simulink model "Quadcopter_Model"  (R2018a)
settings: Solver=VariableStepAuto  StartTime=0.0  StopTime=runtime  FixedStep=0.001  RelTol=1e-3
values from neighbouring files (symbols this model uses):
  delta_T = [ 0,  0,  9.404e-04 ]    [modelParameters.m]    (also in rich_params.m = [ 0,  0,  1.176e-04 ])
  g = 9.81    [modelParameters.m]    (also in rich_params.m)
  height_controlled_o = (((Rm*If        + (((omega0_o * 2 * Rm * Kv * Kq      * Kd + 1)^2) - 1)/(4* Rm*Kv^2*Kq      * Kd))/Vb)*(Pmax - Pmin) + Pmin)    [modelParameters.m]    (also in rich_params.m)
  If = 0.3836    [modelParameters.m]    (also in rich_params.m = 0.39)
  Jreq = 4.2012e-05    [modelParameters.m]    (also in rich_params.m = 1.376e-05)
  Jxx = 0.0110    (= 0.011)    [modelParameters.m]    (also in rich_params.m = 0.0081)
  Jyy = 0.0116    [modelParameters.m]    (also in rich_params.m = 0.0074)
  Jzz = 0.0223    [modelParameters.m]    (also in rich_params.m = 0.0135)
  Kd = 1.4852e-07    [modelParameters.m]    (also in rich_params.m = 5.194e-07)
  Kh = 3.4574e-04    (= 0.00034574)    [modelParameters.m]    (also in rich_params.m)
  Kq = 96.3422    [modelParameters.m]    (also in rich_params.m = 110)
  Kt = 1.2007e-05    [modelParameters.m]    (also in rich_params.m = 7.3956e-06)
  Kv = 96.3422    [modelParameters.m]    (also in rich_params.m = 110)
  m = 1.216    [modelParameters.m]    (also in rich_params.m = 0.656)
  omega0_o = sqrt((m*g)/(4*Kt))    [modelParameters.m]    (also in rich_params.m)
  omega1_o = sqrt((m*g)/(4*Kt))    [modelParameters.m]    (also in rich_params.m)
  omega2_o = sqrt((m*g)/(4*Kt))    [modelParameters.m]    (also in rich_params.m)
  omega3_o = sqrt((m*g)/(4*Kt))    [modelParameters.m]    (also in rich_params.m)
  pitch_o = 0    [modelParameters.m]    (also in rich_params.m)
  pitchrate_o = 0    [modelParameters.m]    (also in rich_params.m)
  Pmax = 1    [modelParameters.m]    (also in rich_params.m)
  Pmin = 0    [modelParameters.m]    (also in rich_params.m)
  r_oc = [ 0 ; 0 ; 0 ]    [modelParameters.m]    (also in rich_params.m)
  rhx = 0.16    [modelParameters.m]    (also in rich_params.m = 0.115)
  rhy = 0.16    [modelParameters.m]    (also in rich_params.m = 0.115)
  rhz = 0.03    [modelParameters.m]    (also in rich_params.m = 0.04)
  Rm = 0.235    [modelParameters.m]    (also in rich_params.m = 0.19)
  roll_o = 0    [modelParameters.m]    (also in rich_params.m)
  rollrate_o = 0    [modelParameters.m]    (also in rich_params.m)
  signal_mixer = [ 1, -1, -1, -1    [modelParameters.m]    (also in rich_params.m)
  Tc = 0.01    [modelParameters.m]    (also in rich_params.m)
  Tq = 0.005    [modelParameters.m]    (also in rich_params.m)
  Vb = 12.3    [modelParameters.m]    (also in rich_params.m = 11.4)
  x_controlled_o = 0    [modelParameters.m]    (also in rich_params.m)
  x_o = 0    [modelParameters.m]    (also in rich_params.m)
  x_vel_o = 0    [modelParameters.m]    (also in rich_params.m)
  y_controlled_o = 0    [modelParameters.m]    (also in rich_params.m)
  y_o = 0    [modelParameters.m]    (also in rich_params.m)
  y_vel_o = 0    [modelParameters.m]    (also in rich_params.m)
  yaw_controlled_o = 0    [modelParameters.m]    (also in rich_params.m)
  yaw_o = 0    [modelParameters.m]    (also in rich_params.m)
  yawrate_o = 0    [modelParameters.m]    (also in rich_params.m)
  z_o = 0    [modelParameters.m]    (also in rich_params.m)
  z_vel_o = 0    [modelParameters.m]    (also in rich_params.m)
undefined symbols (not defined in the file or in its folder): lqr_K
libraries: simulink x16, Derivative x13, dsparch4 x3, vrlib x1
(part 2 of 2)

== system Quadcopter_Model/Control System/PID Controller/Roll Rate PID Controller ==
  rollrate_error : Inport
  rollrate : Inport  Port=2
  Add : Sum  Inputs=+-
  Discrete D Controller : Derivative/Discrete D Controller  Kd=Kd  a=a
  Discrete PI Controller : simulink/Continuous/PID Controller  Controller=PI  TimeDomain=Discrete-time  SampleTime=Ts  IntegratorMethod=Forward Euler  FilterMethod=Forward Euler  Form=Parallel  UseFilter=on  ControllerParametersSource=internal  P=Kp  I=Ki  D=0  N=100  InitialConditionSource=internal  InitialConditionForIntegrator=0  InitialConditionForFilter=0  ExternalReset=none  LimitOutput=off  UpperSaturationLimit=inf  LowerSaturationLimit=-inf  LinearizeAsGain=off  AntiWindupMode=none  Kb=1  TrackingMode=off  Kt=1  PParamMin=[]  PParamMax=[]  IParamMin=[]  IParamMax=[]  DParamMin=[]  DParamMax=[]  NParamMin=[]  NParamMax=[]  KbParamMin=[]  KbParamMax=[]  KtParamMin=[]  KtParamMax=[]  POutMin=[]  POutMax=[]  IOutMin=[]  IOutMax=[]  DOutMin=[]  DOutMax=[]  NOutMin=[]  NOutMax=[]  KbOutMin=[]  KbOutMax=[]  KtOutMin=[]  KtOutMax=[]  IntegratorOutMin=[]  IntegratorOutMax=[]  FilterOutMin=[]  FilterOutMax=[]  SumOutMin=[]  SumOutMax=[]  SumI1OutMin=[]  SumI1OutMax=[]  SumI2OutMin=[]  SumI2OutMax=[]  SumI3OutMin=[]  SumI3OutMax=[]  SumDOutMin=[]  SumDOutMax=[]  SaturationOutMin=[]  SaturationOutMax=[]  IntegratorContinuousStateAttributes=''  IntegratorStateMustResolveToSignalObject=off  IntegratorRTWStateStorageClass=Auto  FilterContinuousStateAttributes=''  FilterStateMustResolveToSignalObject=off  FilterRTWStateStorageClass=Auto  DifferentiatorICPrevScaledInput=0  DifferentiatorOutMin=[]  DifferentiatorOutMax=[]  FilterDiffOutCoefMin=[]  FilterDiffOutCoefMax=[]  SumDenOutMin=[]  SumDenOutMax=[]  SumNumOutMin=[]  SumNumOutMax=[]  ReciprocalOutMin=[]  ReciprocalOutMax=[]  DivideOutMin=[]  DivideOutMax=[]  TunerSelectOption=Transfer Function Based (PID Tuner App)
  y_motor_command : Outport
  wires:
  rollrate/1 -> Discrete D Controller/1
  rollrate_error/1 -> Discrete PI Controller/1
  Discrete PI Controller/1 -> Add/1
  Discrete D Controller/1 -> Add/2
  Add/1 -> y_motor_command/1

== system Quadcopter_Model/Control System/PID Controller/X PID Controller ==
  x_error : Inport
  x_pos : Inport  Port=2
  Add : Sum  Inputs=+-
  Discrete D Controller : Derivative/Discrete D Controller  Kd=Kd  a=a
  Discrete PI Controller : simulink/Continuous/PID Controller  Controller=PI  TimeDomain=Discrete-time  SampleTime=Ts  IntegratorMethod=Forward Euler  FilterMethod=Forward Euler  Form=Parallel  UseFilter=on  ControllerParametersSource=internal  P=Kp  I=Ki  D=0  N=100  InitialConditionSource=internal  InitialConditionForIntegrator=0  InitialConditionForFilter=0  ExternalReset=none  LimitOutput=off  UpperSaturationLimit=inf  LowerSaturationLimit=-inf  LinearizeAsGain=off  AntiWindupMode=none  Kb=1  TrackingMode=off  Kt=1  PParamMin=[]  PParamMax=[]  IParamMin=[]  IParamMax=[]  DParamMin=[]  DParamMax=[]  NParamMin=[]  NParamMax=[]  KbParamMin=[]  KbParamMax=[]  KtParamMin=[]  KtParamMax=[]  POutMin=[]  POutMax=[]  IOutMin=[]  IOutMax=[]  DOutMin=[]  DOutMax=[]  NOutMin=[]  NOutMax=[]  KbOutMin=[]  KbOutMax=[]  KtOutMin=[]  KtOutMax=[]  IntegratorOutMin=[]  IntegratorOutMax=[]  FilterOutMin=[]  FilterOutMax=[]  SumOutMin=[]  SumOutMax=[]  SumI1OutMin=[]  SumI1OutMax=[]  SumI2OutMin=[]  SumI2OutMax=[]  SumI3OutMin=[]  SumI3OutMax=[]  SumDOutMin=[]  SumDOutMax=[]  SaturationOutMin=[]  SaturationOutMax=[]  IntegratorContinuousStateAttributes=''  IntegratorStateMustResolveToSignalObject=off  IntegratorRTWStateStorageClass=Auto  FilterContinuousStateAttributes=''  FilterStateMustResolveToSignalObject=off  FilterRTWStateStorageClass=Auto  DifferentiatorICPrevScaledInput=0  DifferentiatorOutMin=[]  DifferentiatorOutMax=[]  FilterDiffOutCoefMin=[]  FilterDiffOutCoefMax=[]  SumDenOutMin=[]  SumDenOutMax=[]  SumNumOutMin=[]  SumNumOutMax=[]  ReciprocalOutMin=[]  ReciprocalOutMax=[]  DivideOutMin=[]  DivideOutMax=[]  TunerSelectOption=Transfer Function Based (PID Tuner App)
  pitch_setpoint : Outport
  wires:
  x_pos/1 -> Discrete D Controller/1
  x_error/1 -> Discrete PI Controller/1
  Discrete PI Controller/1 -> Add/1
  Discrete D Controller/1 -> Add/2
  Add/1 -> pitch_setpoint/1

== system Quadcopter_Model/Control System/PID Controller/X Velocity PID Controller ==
  x_vel_error : Inport
  x_vel : Inport  Port=2
  Add : Sum  Inputs=+-
  Discrete D Controller : Derivative/Discrete D Controller  Kd=Kd  a=a
  Discrete PI Controller : simulink/Continuous/PID Controller  Controller=PI  TimeDomain=Discrete-time  SampleTime=Ts  IntegratorMethod=Forward Euler  FilterMethod=Forward Euler  Form=Parallel  UseFilter=on  ControllerParametersSource=internal  P=Kp  I=Ki  D=0  N=100  InitialConditionSource=internal  InitialConditionForIntegrator=0  InitialConditionForFilter=0  ExternalReset=none  LimitOutput=off  UpperSaturationLimit=inf  LowerSaturationLimit=-inf  LinearizeAsGain=off  AntiWindupMode=none  Kb=1  TrackingMode=off  Kt=1  PParamMin=[]  PParamMax=[]  IParamMin=[]  IParamMax=[]  DParamMin=[]  DParamMax=[]  NParamMin=[]  NParamMax=[]  KbParamMin=[]  KbParamMax=[]  KtParamMin=[]  KtParamMax=[]  POutMin=[]  POutMax=[]  IOutMin=[]  IOutMax=[]  DOutMin=[]  DOutMax=[]  NOutMin=[]  NOutMax=[]  KbOutMin=[]  KbOutMax=[]  KtOutMin=[]  KtOutMax=[]  IntegratorOutMin=[]  IntegratorOutMax=[]  FilterOutMin=[]  FilterOutMax=[]  SumOutMin=[]  SumOutMax=[]  SumI1OutMin=[]  SumI1OutMax=[]  SumI2OutMin=[]  SumI2OutMax=[]  SumI3OutMin=[]  SumI3OutMax=[]  SumDOutMin=[]  SumDOutMax=[]  SaturationOutMin=[]  SaturationOutMax=[]  IntegratorContinuousStateAttributes=''  IntegratorStateMustResolveToSignalObject=off  IntegratorRTWStateStorageClass=Auto  FilterContinuousStateAttributes=''  FilterStateMustResolveToSignalObject=off  FilterRTWStateStorageClass=Auto  DifferentiatorICPrevScaledInput=0  DifferentiatorOutMin=[]  DifferentiatorOutMax=[]  FilterDiffOutCoefMin=[]  FilterDiffOutCoefMax=[]  SumDenOutMin=[]  SumDenOutMax=[]  SumNumOutMin=[]  SumNumOutMax=[]  ReciprocalOutMin=[]  ReciprocalOutMax=[]  DivideOutMin=[]  DivideOutMax=[]  TunerSelectOption=Transfer Function Based (PID Tuner App)
  pitch_setpoint : Outport
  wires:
  x_vel/1 -> Discrete D Controller/1
  x_vel_error/1 -> Discrete PI Controller/1
  Discrete PI Controller/1 -> Add/1
  Discrete D Controller/1 -> Add/2
  Add/1 -> pitch_setpoint/1

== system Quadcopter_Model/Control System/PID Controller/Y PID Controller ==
  y_error : Inport
  y_pos : Inport  Port=2
  Add : Sum  Inputs=+-
  Discrete D Controller : Derivative/Discrete D Controller  Kd=Kd  a=a
  Discrete PI Controller : simulink/Continuous/PID Controller  Controller=PI  TimeDomain=Discrete-time  SampleTime=Ts  IntegratorMethod=Forward Euler  FilterMethod=Forward Euler  Form=Parallel  UseFilter=on  ControllerParametersSource=internal  P=Kp  I=Ki  D=0  N=100  InitialConditionSource=internal  InitialConditionForIntegrator=0  InitialConditionForFilter=0  ExternalReset=none  LimitOutput=off  UpperSaturationLimit=inf  LowerSaturationLimit=-inf  LinearizeAsGain=off  AntiWindupMode=none  Kb=1  TrackingMode=off  Kt=1  PParamMin=[]  PParamMax=[]  IParamMin=[]  IParamMax=[]  DParamMin=[]  DParamMax=[]  NParamMin=[]  NParamMax=[]  KbParamMin=[]  KbParamMax=[]  KtParamMin=[]  KtParamMax=[]  POutMin=[]  POutMax=[]  IOutMin=[]  IOutMax=[]  DOutMin=[]  DOutMax=[]  NOutMin=[]  NOutMax=[]  KbOutMin=[]  KbOutMax=[]  KtOutMin=[]  KtOutMax=[]  IntegratorOutMin=[]  IntegratorOutMax=[]  FilterOutMin=[]  FilterOutMax=[]  SumOutMin=[]  SumOutMax=[]  SumI1OutMin=[]  SumI1OutMax=[]  SumI2OutMin=[]  SumI2OutMax=[]  SumI3OutMin=[]  SumI3OutMax=[]  SumDOutMin=[]  SumDOutMax=[]  SaturationOutMin=[]  SaturationOutMax=[]  IntegratorContinuousStateAttributes=''  IntegratorStateMustResolveToSignalObject=off  IntegratorRTWStateStorageClass=Auto  FilterContinuousStateAttributes=''  FilterStateMustResolveToSignalObject=off  FilterRTWStateStorageClass=Auto  DifferentiatorICPrevScaledInput=0  DifferentiatorOutMin=[]  DifferentiatorOutMax=[]  FilterDiffOutCoefMin=[]  FilterDiffOutCoefMax=[]  SumDenOutMin=[]  SumDenOutMax=[]  SumNumOutMin=[]  SumNumOutMax=[]  ReciprocalOutMin=[]  ReciprocalOutMax=[]  DivideOutMin=[]  DivideOutMax=[]  TunerSelectOption=Transfer Function Based (PID Tuner App)
  roll_setpoint : Outport
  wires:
  y_pos/1 -> Discrete D Controller/1
  y_error/1 -> Discrete PI Controller/1
  Discrete PI Controller/1 -> Add/1
  Discrete D Controller/1 -> Add/2
  Add/1 -> roll_setpoint/1

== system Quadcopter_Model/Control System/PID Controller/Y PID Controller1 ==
  y_error : Inport
  y_pos : Inport  Port=2
  Add : Sum  Inputs=+-
  Discrete D Controller : Derivative/Discrete D Controller  Kd=Kd  a=a
  Discrete PI Controller : simulink/Continuous/PID Controller  Controller=PI  TimeDomain=Discrete-time  SampleTime=Ts  IntegratorMethod=Forward Euler  FilterMethod=Forward Euler  Form=Parallel  UseFilter=on  ControllerParametersSource=internal  P=Kp  I=Ki  D=0  N=100  InitialConditionSource=internal  InitialConditionForIntegrator=0  InitialConditionForFilter=0  ExternalReset=none  LimitOutput=off  UpperSaturationLimit=inf  LowerSaturationLimit=-inf  LinearizeAsGain=off  AntiWindupMode=none  Kb=1  TrackingMode=off  Kt=1  PParamMin=[]  PParamMax=[]  IParamMin=[]  IParamMax=[]  DParamMin=[]  DParamMax=[]  NParamMin=[]  NParamMax=[]  KbParamMin=[]  KbParamMax=[]  KtParamMin=[]  KtParamMax=[]  POutMin=[]  POutMax=[]  IOutMin=[]  IOutMax=[]  DOutMin=[]  DOutMax=[]  NOutMin=[]  NOutMax=[]  KbOutMin=[]  KbOutMax=[]  KtOutMin=[]  KtOutMax=[]  IntegratorOutMin=[]  IntegratorOutMax=[]  FilterOutMin=[]  FilterOutMax=[]  SumOutMin=[]  SumOutMax=[]  SumI1OutMin=[]  SumI1OutMax=[]  SumI2OutMin=[]  SumI2OutMax=[]  SumI3OutMin=[]  SumI3OutMax=[]  SumDOutMin=[]  SumDOutMax=[]  SaturationOutMin=[]  SaturationOutMax=[]  IntegratorContinuousStateAttributes=''  IntegratorStateMustResolveToSignalObject=off  IntegratorRTWStateStorageClass=Auto  FilterContinuousStateAttributes=''  FilterStateMustResolveToSignalObject=off  FilterRTWStateStorageClass=Auto  DifferentiatorICPrevScaledInput=0  DifferentiatorOutMin=[]  DifferentiatorOutMax=[]  FilterDiffOutCoefMin=[]  FilterDiffOutCoefMax=[]  SumDenOutMin=[]  SumDenOutMax=[]  SumNumOutMin=[]  SumNumOutMax=[]  ReciprocalOutMin=[]  ReciprocalOutMax=[]  DivideOutMin=[]  DivideOutMax=[]  TunerSelectOption=Transfer Function Based (PID Tuner App)
  y_vel_setpoint : Outport
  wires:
  y_pos/1 -> Discrete D Controller/1
  y_error/1 -> Discrete PI Controller/1
  Discrete PI Controller/1 -> Add/1
  Discrete D Controller/1 -> Add/2
  Add/1 -> y_vel_setpoint/1

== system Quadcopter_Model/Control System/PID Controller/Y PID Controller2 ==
  x_error : Inport
  x_pos : Inport  Port=2
  Add : Sum  Inputs=+-
  Discrete D Controller : Derivative/Discrete D Controller  Kd=Kd  a=a
  Discrete PI Controller : simulink/Continuous/PID Controller  Controller=PI  TimeDomain=Discrete-time  SampleTime=Ts  IntegratorMethod=Forward Euler  FilterMethod=Forward Euler  Form=Parallel  UseFilter=on  ControllerParametersSource=internal  P=Kp  I=Ki  D=0  N=100  InitialConditionSource=internal  InitialConditionForIntegrator=0  InitialConditionForFilter=0  ExternalReset=none  LimitOutput=off  UpperSaturationLimit=inf  LowerSaturationLimit=-inf  LinearizeAsGain=off  AntiWindupMode=none  Kb=1  TrackingMode=off  Kt=1  PParamMin=[]  PParamMax=[]  IParamMin=[]  IParamMax=[]  DParamMin=[]  DParamMax=[]  NParamMin=[]  NParamMax=[]  KbParamMin=[]  KbParamMax=[]  KtParamMin=[]  KtParamMax=[]  POutMin=[]  POutMax=[]  IOutMin=[]  IOutMax=[]  DOutMin=[]  DOutMax=[]  NOutMin=[]  NOutMax=[]  KbOutMin=[]  KbOutMax=[]  KtOutMin=[]  KtOutMax=[]  IntegratorOutMin=[]  IntegratorOutMax=[]  FilterOutMin=[]  FilterOutMax=[]  SumOutMin=[]  SumOutMax=[]  SumI1OutMin=[]  SumI1OutMax=[]  SumI2OutMin=[]  SumI2OutMax=[]  SumI3OutMin=[]  SumI3OutMax=[]  SumDOutMin=[]  SumDOutMax=[]  SaturationOutMin=[]  SaturationOutMax=[]  IntegratorContinuousStateAttributes=''  IntegratorStateMustResolveToSignalObject=off  IntegratorRTWStateStorageClass=Auto  FilterContinuousStateAttributes=''  FilterStateMustResolveToSignalObject=off  FilterRTWStateStorageClass=Auto  DifferentiatorICPrevScaledInput=0  DifferentiatorOutMin=[]  DifferentiatorOutMax=[]  FilterDiffOutCoefMin=[]  FilterDiffOutCoefMax=[]  SumDenOutMin=[]  SumDenOutMax=[]  SumNumOutMin=[]  SumNumOutMax=[]  ReciprocalOutMin=[]  ReciprocalOutMax=[]  DivideOutMin=[]  DivideOutMax=[]  TunerSelectOption=Transfer Function Based (PID Tuner App)
  x_vel_setpoint : Outport
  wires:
  x_pos/1 -> Discrete D Controller/1
  x_error/1 -> Discrete PI Controller/1
  Discrete PI Controller/1 -> Add/1
  Discrete D Controller/1 -> Add/2
  Add/1 -> x_vel_setpoint/1

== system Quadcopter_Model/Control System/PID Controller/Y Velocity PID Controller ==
  y_error : Inport
  y_pos : Inport  Port=2
  Add : Sum  Inputs=+-
  Discrete D Controller : Derivative/Discrete D Controller  Kd=Kd  a=a
  Discrete PI Controller : simulink/Continuous/PID Controller  Controller=PI  TimeDomain=Discrete-time  SampleTime=Ts  IntegratorMethod=Forward Euler  FilterMethod=Forward Euler  Form=Parallel  UseFilter=on  ControllerParametersSource=internal  P=Kp  I=Ki  D=0  N=100  InitialConditionSource=internal  InitialConditionForIntegrator=0  InitialConditionForFilter=0  ExternalReset=none  LimitOutput=off  UpperSaturationLimit=inf  LowerSaturationLimit=-inf  LinearizeAsGain=off  AntiWindupMode=none  Kb=1  TrackingMode=off  Kt=1  PParamMin=[]  PParamMax=[]  IParamMin=[]  IParamMax=[]  DParamMin=[]  DParamMax=[]  NParamMin=[]  NParamMax=[]  KbParamMin=[]  KbParamMax=[]  KtParamMin=[]  KtParamMax=[]  POutMin=[]  POutMax=[]  IOutMin=[]  IOutMax=[]  DOutMin=[]  DOutMax=[]  NOutMin=[]  NOutMax=[]  KbOutMin=[]  KbOutMax=[]  KtOutMin=[]  KtOutMax=[]  IntegratorOutMin=[]  IntegratorOutMax=[]  FilterOutMin=[]  FilterOutMax=[]  SumOutMin=[]  SumOutMax=[]  SumI1OutMin=[]  SumI1OutMax=[]  SumI2OutMin=[]  SumI2OutMax=[]  SumI3OutMin=[]  SumI3OutMax=[]  SumDOutMin=[]  SumDOutMax=[]  SaturationOutMin=[]  SaturationOutMax=[]  IntegratorContinuousStateAttributes=''  IntegratorStateMustResolveToSignalObject=off  IntegratorRTWStateStorageClass=Auto  FilterContinuousStateAttributes=''  FilterStateMustResolveToSignalObject=off  FilterRTWStateStorageClass=Auto  DifferentiatorICPrevScaledInput=0  DifferentiatorOutMin=[]  DifferentiatorOutMax=[]  FilterDiffOutCoefMin=[]  FilterDiffOutCoefMax=[]  SumDenOutMin=[]  SumDenOutMax=[]  SumNumOutMin=[]  SumNumOutMax=[]  ReciprocalOutMin=[]  ReciprocalOutMax=[]  DivideOutMin=[]  DivideOutMax=[]  TunerSelectOption=Transfer Function Based (PID Tuner App)
  roll_setpoint : Outport
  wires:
  y_pos/1 -> Discrete D Controller/1
  y_error/1 -> Discrete PI Controller/1
  Discrete PI Controller/1 -> Add/1
  Discrete D Controller/1 -> Add/2
  Add/1 -> roll_setpoint/1

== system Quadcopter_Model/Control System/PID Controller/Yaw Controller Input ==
  note: 1) Add Subsystem or Model blocks as valid variant choices. 2) You cannot connect blocks at this level. At simulation, connectivity is automatically determined, based on the active variant and port name matching.
  yaw_error_model : Inport
  yaw_angle_model : Inport  Port=2
  Feedback : Subsystem  VariantControl=logAnalysisToggle==0
  yaw error : Subsystem  VariantControl=logAnalysisToggle==1
  yaw_error : Outport
  yaw_angle : Outport  Port=2

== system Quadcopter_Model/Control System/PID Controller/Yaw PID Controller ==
  yaw_error : Inport
  yaw_angle : Inport  Port=2
  Add : Sum  Inputs=+-
  Discrete D Controller : Derivative/Discrete D Controller  Kd=Kd  a=a
  Discrete PI Controller : simulink/Continuous/PID Controller  Controller=PI  TimeDomain=Discrete-time  SampleTime=Ts  IntegratorMethod=Forward Euler  FilterMethod=Forward Euler  Form=Parallel  UseFilter=on  ControllerParametersSource=internal  P=Kp  I=Ki  D=0  N=100  InitialConditionSource=internal  InitialConditionForIntegrator=0  InitialConditionForFilter=0  ExternalReset=none  LimitOutput=off  UpperSaturationLimit=inf  LowerSaturationLimit=-inf  LinearizeAsGain=off  AntiWindupMode=none  Kb=1  TrackingMode=off  Kt=1  PParamMin=[]  PParamMax=[]  IParamMin=[]  IParamMax=[]  DParamMin=[]  DParamMax=[]  NParamMin=[]  NParamMax=[]  KbParamMin=[]  KbParamMax=[]  KtParamMin=[]  KtParamMax=[]  POutMin=[]  POutMax=[]  IOutMin=[]  IOutMax=[]  DOutMin=[]  DOutMax=[]  NOutMin=[]  NOutMax=[]  KbOutMin=[]  KbOutMax=[]  KtOutMin=[]  KtOutMax=[]  IntegratorOutMin=[]  IntegratorOutMax=[]  FilterOutMin=[]  FilterOutMax=[]  SumOutMin=[]  SumOutMax=[]  SumI1OutMin=[]  SumI1OutMax=[]  SumI2OutMin=[]  SumI2OutMax=[]  SumI3OutMin=[]  SumI3OutMax=[]  SumDOutMin=[]  SumDOutMax=[]  SaturationOutMin=[]  SaturationOutMax=[]  IntegratorContinuousStateAttributes=''  IntegratorStateMustResolveToSignalObject=off  IntegratorRTWStateStorageClass=Auto  FilterContinuousStateAttributes=''  FilterStateMustResolveToSignalObject=off  FilterRTWStateStorageClass=Auto  DifferentiatorICPrevScaledInput=0  DifferentiatorOutMin=[]  DifferentiatorOutMax=[]  FilterDiffOutCoefMin=[]  FilterDiffOutCoefMax=[]  SumDenOutMin=[]  SumDenOutMax=[]  SumNumOutMin=[]  SumNumOutMax=[]  ReciprocalOutMin=[]  ReciprocalOutMax=[]  DivideOutMin=[]  DivideOutMax=[]  TunerSelectOption=Transfer Function Based (PID Tuner App)
  yawrate_setpoint : Outport
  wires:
  yaw_angle/1 -> Discrete D Controller/1
  yaw_error/1 -> Discrete PI Controller/1
  Discrete PI Controller/1 -> Add/1
  Discrete D Controller/1 -> Add/2
  Add/1 -> yawrate_setpoint/1

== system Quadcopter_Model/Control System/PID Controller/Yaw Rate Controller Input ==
  note: 1) Add Subsystem or Model blocks as valid variant choices. 2) You cannot connect blocks at this level. At simulation, connectivity is automatically determined, based on the active variant and port name matching.
  yawrate_error_model : Inport
  yawrate_model : Inport  Port=2
  Feedback : Subsystem  VariantControl=logAnalysisToggle==0
  yawrate error : Subsystem  VariantControl=logAnalysisToggle==1
  yawrate_error : Outport
  yawrate : Outport  Port=2

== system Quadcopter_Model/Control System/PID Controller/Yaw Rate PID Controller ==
  yawrate_error : Inport
  yawrate : Inport  Port=2
  Add : Sum  Inputs=+-
  Discrete D Controller : Derivative/Discrete D Controller  Kd=Kd  a=a
  Discrete PI Controller : simulink/Continuous/PID Controller  Controller=PI  TimeDomain=Discrete-time  SampleTime=Ts  IntegratorMethod=Forward Euler  FilterMethod=Forward Euler  Form=Parallel  UseFilter=on  ControllerParametersSource=internal  P=Kp  I=Ki  D=0  N=100  InitialConditionSource=internal  InitialConditionForIntegrator=0  InitialConditionForFilter=0  ExternalReset=none  LimitOutput=off  UpperSaturationLimit=inf  LowerSaturationLimit=-inf  LinearizeAsGain=off  AntiWindupMode=none  Kb=1  TrackingMode=off  Kt=1  PParamMin=[]  PParamMax=[]  IParamMin=[]  IParamMax=[]  DParamMin=[]  DParamMax=[]  NParamMin=[]  NParamMax=[]  KbParamMin=[]  KbParamMax=[]  KtParamMin=[]  KtParamMax=[]  POutMin=[]  POutMax=[]  IOutMin=[]  IOutMax=[]  DOutMin=[]  DOutMax=[]  NOutMin=[]  NOutMax=[]  KbOutMin=[]  KbOutMax=[]  KtOutMin=[]  KtOutMax=[]  IntegratorOutMin=[]  IntegratorOutMax=[]  FilterOutMin=[]  FilterOutMax=[]  SumOutMin=[]  SumOutMax=[]  SumI1OutMin=[]  SumI1OutMax=[]  SumI2OutMin=[]  SumI2OutMax=[]  SumI3OutMin=[]  SumI3OutMax=[]  SumDOutMin=[]  SumDOutMax=[]  SaturationOutMin=[]  SaturationOutMax=[]  IntegratorContinuousStateAttributes=''  IntegratorStateMustResolveToSignalObject=off  IntegratorRTWStateStorageClass=Auto  FilterContinuousStateAttributes=''  FilterStateMustResolveToSignalObject=off  FilterRTWStateStorageClass=Auto  DifferentiatorICPrevScaledInput=0  DifferentiatorOutMin=[]  DifferentiatorOutMax=[]  FilterDiffOutCoefMin=[]  FilterDiffOutCoefMax=[]  SumDenOutMin=[]  SumDenOutMax=[]  SumNumOutMin=[]  SumNumOutMax=[]  ReciprocalOutMin=[]  ReciprocalOutMax=[]  DivideOutMin=[]  DivideOutMax=[]  TunerSelectOption=Transfer Function Based (PID Tuner App)
  yaw_motor_command : Outport
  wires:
  yawrate/1 -> Discrete D Controller/1
  yawrate_error/1 -> Discrete PI Controller/1
  Discrete PI Controller/1 -> Add/1
  Discrete D Controller/1 -> Add/2
  Add/1 -> yaw_motor_command/1

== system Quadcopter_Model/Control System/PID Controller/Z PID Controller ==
  z_error : Inport
  z_pos : Inport  Port=2
  Add : Sum  Inputs=+-
  Discrete D Controller : Derivative/Discrete D Controller  Kd=Kd  a=a
  Discrete PI Controller : simulink/Continuous/PID Controller  Controller=PI  TimeDomain=Discrete-time  SampleTime=Ts  IntegratorMethod=Forward Euler  FilterMethod=Forward Euler  Form=Parallel  UseFilter=on  ControllerParametersSource=internal  P=Kp  I=Ki  D=0  N=100  InitialConditionSource=internal  InitialConditionForIntegrator=0  InitialConditionForFilter=0  ExternalReset=none  LimitOutput=off  UpperSaturationLimit=inf  LowerSaturationLimit=-inf  LinearizeAsGain=off  AntiWindupMode=none  Kb=1  TrackingMode=off  Kt=1  PParamMin=[]  PParamMax=[]  IParamMin=[]  IParamMax=[]  DParamMin=[]  DParamMax=[]  NParamMin=[]  NParamMax=[]  KbParamMin=[]  KbParamMax=[]  KtParamMin=[]  KtParamMax=[]  POutMin=[]  POutMax=[]  IOutMin=[]  IOutMax=[]  DOutMin=[]  DOutMax=[]  NOutMin=[]  NOutMax=[]  KbOutMin=[]  KbOutMax=[]  KtOutMin=[]  KtOutMax=[]  IntegratorOutMin=[]  IntegratorOutMax=[]  FilterOutMin=[]  FilterOutMax=[]  SumOutMin=[]  SumOutMax=[]  SumI1OutMin=[]  SumI1OutMax=[]  SumI2OutMin=[]  SumI2OutMax=[]  SumI3OutMin=[]  SumI3OutMax=[]  SumDOutMin=[]  SumDOutMax=[]  SaturationOutMin=[]  SaturationOutMax=[]  IntegratorContinuousStateAttributes=''  IntegratorStateMustResolveToSignalObject=off  IntegratorRTWStateStorageClass=Auto  FilterContinuousStateAttributes=''  FilterStateMustResolveToSignalObject=off  FilterRTWStateStorageClass=Auto  DifferentiatorICPrevScaledInput=0  DifferentiatorOutMin=[]  DifferentiatorOutMax=[]  FilterDiffOutCoefMin=[]  FilterDiffOutCoefMax=[]  SumDenOutMin=[]  SumDenOutMax=[]  SumNumOutMin=[]  SumNumOutMax=[]  ReciprocalOutMin=[]  ReciprocalOutMax=[]  DivideOutMin=[]  DivideOutMax=[]  TunerSelectOption=Transfer Function Based (PID Tuner App)
  z_motor_command : Outport
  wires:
  z_pos/1 -> Discrete D Controller/1
  z_error/1 -> Discrete PI Controller/1
  Discrete PI Controller/1 -> Add/1
  Discrete D Controller/1 -> Add/2
  Add/1 -> z_motor_command/1

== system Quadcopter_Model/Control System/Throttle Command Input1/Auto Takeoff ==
  height_controlled_o : Constant  Value=0.45  SampleTime=Tc
  z_command : Outport
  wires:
  height_controlled_o/1 -> z_command/1

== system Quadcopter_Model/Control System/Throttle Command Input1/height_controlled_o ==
  height_controlled_o : Constant  Value=height_controlled_o  SampleTime=Tc
  z_command : Outport
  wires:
  height_controlled_o/1 -> z_command/1

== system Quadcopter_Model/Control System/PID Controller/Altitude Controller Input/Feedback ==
  z_error_model : Inport
  z_position_model : Inport  Port=2
  z_error : Outport
  z_position : Outport  Port=2
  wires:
  z_error_model/1 -> z_error/1
  z_position_model/1 -> z_position/1

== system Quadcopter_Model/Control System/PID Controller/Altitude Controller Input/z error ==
  From Workspace1 : FromWorkspace  VariableName=z_position  SampleTime=Tc  Interpolate=off  OutputAfterFinalValue=Holding final value
  From Workspace6 : FromWorkspace  VariableName=z_error  SampleTime=Tc  Interpolate=off  OutputAfterFinalValue=Holding final value
  z_error : Outport
  z_position : Outport  Port=2
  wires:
  From Workspace6/1 -> z_error/1
  From Workspace1/1 -> z_position/1

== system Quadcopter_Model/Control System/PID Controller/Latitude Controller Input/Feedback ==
  x_error_model : Inport
  x_position_model : Inport  Port=2
  x_error : Outport
  x_position : Outport  Port=2
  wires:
  x_error_model/1 -> x_error/1
  x_position_model/1 -> x_position/1

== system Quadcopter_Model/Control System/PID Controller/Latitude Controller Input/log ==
  From Workspace : FromWorkspace  VariableName=x_error  SampleTime=Tc  Interpolate=off  OutputAfterFinalValue=Holding final value
  From Workspace1 : FromWorkspace  VariableName=x_position  SampleTime=Tc  Interpolate=off  OutputAfterFinalValue=Holding final value
  x_error : Outport
  x_position : Outport  Port=2
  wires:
  From Workspace/1 -> x_error/1
  From Workspace1/1 -> x_position/1

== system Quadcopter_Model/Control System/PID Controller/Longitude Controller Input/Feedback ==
  y_error_model : Inport
  y_position_model : Inport  Port=2
  y_error : Outport
  y_position : Outport  Port=2
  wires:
  y_error_model/1 -> y_error/1
  y_position_model/1 -> y_position/1

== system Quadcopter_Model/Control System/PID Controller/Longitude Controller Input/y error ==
  From Workspace1 : FromWorkspace  VariableName=y_position  SampleTime=Tc  Interpolate=off  OutputAfterFinalValue=Holding final value
  From Workspace3 : FromWorkspace  VariableName=y_error  SampleTime=Tc  Interpolate=off  OutputAfterFinalValue=Holding final value
  y_error : Outport
  y_position : Outport  Port=2
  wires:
  From Workspace3/1 -> y_error/1
  From Workspace1/1 -> y_position/1

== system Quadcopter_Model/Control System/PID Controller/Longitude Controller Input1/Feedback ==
  y_vel_error_model : Inport
  y_vel_model : Inport  Port=2
  y_vel_error : Outport
  y_vel : Outport  Port=2
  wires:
  y_vel_error_model/1 -> y_vel_error/1
  y_vel_model/1 -> y_vel/1

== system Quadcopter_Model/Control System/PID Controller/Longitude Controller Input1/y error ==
  From Workspace1 : FromWorkspace  VariableName=y_vel  SampleTime=Tc  Interpolate=off  OutputAfterFinalValue=Holding final value
  From Workspace3 : FromWorkspace  VariableName=y_vel_error  SampleTime=Tc  Interpolate=off  OutputAfterFinalValue=Holding final value
  y_vel_error : Outport
  y_vel : Outport  Port=2
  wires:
  From Workspace3/1 -> y_vel_error/1
  From Workspace1/1 -> y_vel/1

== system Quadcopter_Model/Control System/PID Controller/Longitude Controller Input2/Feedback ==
  x_vel_error_model : Inport
  x_vel_model : Inport  Port=2
  x_vel_error : Outport
  x_vel : Outport  Port=2
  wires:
  x_vel_error_model/1 -> x_vel_error/1
  x_vel_model/1 -> x_vel/1

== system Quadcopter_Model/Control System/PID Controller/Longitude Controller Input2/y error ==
  From Workspace1 : FromWorkspace  VariableName=x_vel  SampleTime=Tc  Interpolate=off  OutputAfterFinalValue=Holding final value
  From Workspace3 : FromWorkspace  VariableName=x_vel_error  SampleTime=Tc  Interpolate=off  OutputAfterFinalValue=Holding final value
  x_vel_error : Outport
  x_vel : Outport  Port=2
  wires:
  From Workspace3/1 -> x_vel_error/1
  From Workspace1/1 -> x_vel/1

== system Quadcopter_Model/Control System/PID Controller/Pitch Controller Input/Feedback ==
  pitch_error_model : Inport
  pitch_angle_model : Inport  Port=2
  pitch_error : Outport
  pitch_angle : Outport  Port=2
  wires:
  pitch_error_model/1 -> pitch_error/1
  pitch_angle_model/1 -> pitch_angle/1

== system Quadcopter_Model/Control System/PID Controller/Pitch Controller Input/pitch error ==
  From Workspace : FromWorkspace  VariableName=pitch_error  SampleTime=Tq  Interpolate=off  OutputAfterFinalValue=Holding final value
  From Workspace1 : FromWorkspace  VariableName=pitch_angle  SampleTime=Tq  Interpolate=off  OutputAfterFinalValue=Holding final value
  pitch_error : Outport
  pitch_angle : Outport  Port=2
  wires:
  From Workspace/1 -> pitch_error/1
  From Workspace1/1 -> pitch_angle/1

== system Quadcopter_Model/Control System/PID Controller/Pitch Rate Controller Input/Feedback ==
  pitchrate_error_model : Inport
  pitchrate_model : Inport  Port=2
  pitchrate_error : Outport
  pitchrate : Outport  Port=2
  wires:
  pitchrate_error_model/1 -> pitchrate_error/1
  pitchrate_model/1 -> pitchrate/1

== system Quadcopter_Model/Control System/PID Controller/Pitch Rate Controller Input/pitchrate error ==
  From Workspace1 : FromWorkspace  VariableName=pitchrate  SampleTime=Tq  Interpolate=off  OutputAfterFinalValue=Holding final value
  From Workspace2 : FromWorkspace  VariableName=pitchrate_error  SampleTime=Tq  Interpolate=off  OutputAfterFinalValue=Holding final value
  pitchrate_error : Outport
  pitchrate : Outport  Port=2
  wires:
  From Workspace2/1 -> pitchrate_error/1
  From Workspace1/1 -> pitchrate/1

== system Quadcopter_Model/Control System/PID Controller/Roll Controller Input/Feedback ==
  roll_error_model : Inport
  roll_angle_model : Inport  Port=2
  roll_error : Outport
  roll_angle : Outport  Port=2
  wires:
  roll_error_model/1 -> roll_error/1
  roll_angle_model/1 -> roll_angle/1

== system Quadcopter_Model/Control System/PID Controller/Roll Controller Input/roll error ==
  From Workspace1 : FromWorkspace  VariableName=roll_angle  SampleTime=Tq  Interpolate=off  OutputAfterFinalValue=Holding final value
  From Workspace4 : FromWorkspace  VariableName=roll_error  SampleTime=Tq  Interpolate=off  OutputAfterFinalValue=Holding final value
  roll_error : Outport
  roll_angle : Outport  Port=2
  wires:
  From Workspace4/1 -> roll_error/1
  From Workspace1/1 -> roll_angle/1

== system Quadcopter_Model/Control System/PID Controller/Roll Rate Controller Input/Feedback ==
  rollrate_error_model : Inport
  rollrate_model : Inport  Port=2
  rollrate_error : Outport
  rollrate : Outport  Port=2
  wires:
  rollrate_error_model/1 -> rollrate_error/1
  rollrate_model/1 -> rollrate/1

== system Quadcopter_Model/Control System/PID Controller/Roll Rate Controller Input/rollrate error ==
  From Workspace1 : FromWorkspace  VariableName=rollrate  SampleTime=Tq  Interpolate=off  OutputAfterFinalValue=Holding final value
  From Workspace5 : FromWorkspace  VariableName=rollrate_error  SampleTime=Tq  Interpolate=off  OutputAfterFinalValue=Holding final value
  rollrate_error : Outport
  rollrate : Outport  Port=2
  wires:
  From Workspace5/1 -> rollrate_error/1
  From Workspace1/1 -> rollrate/1

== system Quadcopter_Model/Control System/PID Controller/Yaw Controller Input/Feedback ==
  yaw_error_model : Inport
  yaw_angle_model : Inport  Port=2
  yaw_error : Outport
  yaw_angle : Outport  Port=2
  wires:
  yaw_error_model/1 -> yaw_error/1
  yaw_angle_model/1 -> yaw_angle/1

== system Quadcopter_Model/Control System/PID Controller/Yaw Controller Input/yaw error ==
  From Workspace1 : FromWorkspace  VariableName=yaw_angle  SampleTime=Tc  Interpolate=off  OutputAfterFinalValue=Holding final value
  From Workspace7 : FromWorkspace  VariableName=yaw_error  SampleTime=Tc  Interpolate=off  OutputAfterFinalValue=Holding final value
  yaw_error : Outport
  yaw_angle : Outport  Port=2
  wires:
  From Workspace7/1 -> yaw_error/1
  From Workspace1/1 -> yaw_angle/1

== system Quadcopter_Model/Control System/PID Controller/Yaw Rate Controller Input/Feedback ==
  yawrate_error_model : Inport
  yawrate_model : Inport  Port=2
  yawrate_error : Outport
  yawrate : Outport  Port=2
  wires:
  yawrate_error_model/1 -> yawrate_error/1
  yawrate_model/1 -> yawrate/1

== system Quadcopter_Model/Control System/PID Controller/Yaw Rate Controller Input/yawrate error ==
  From Workspace1 : FromWorkspace  VariableName=yawrate  SampleTime=Tq  Interpolate=off  OutputAfterFinalValue=Holding final value
  From Workspace8 : FromWorkspace  VariableName=yawrate_error  SampleTime=Tq  Interpolate=off  OutputAfterFinalValue=Holding final value
  yawrate_error : Outport
  yawrate : Outport  Port=2
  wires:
  From Workspace8/1 -> yawrate_error/1
  From Workspace1/1 -> yawrate/1

== matlab function Quadcopter_Model/Actuation/Gravity

 ==
function E_Fg = gravity(m, g)

E_Fg = [0; 0; m*g];

== matlab function Quadcopter_Model/Actuation/Lbe





 ==
function E_ro  = linear_body_earth_conversion(B_vo, euler_angles)

euler_rates = zeros(3,1);
E_ro = zeros(3,1);

phi = euler_angles(1);
theta = euler_angles(2);
psi = euler_angles(3);

Leb = [cos(theta)*cos(psi), sin(phi)*sin(theta)*cos(psi)-cos(phi)*sin(psi), cos(phi)*sin(theta)*cos(psi)+sin(phi)*sin(psi); ...
       cos(theta)*sin(psi), sin(phi)*sin(theta)*sin(psi)+cos(phi)*cos(psi), cos(phi)*sin(theta)*sin(psi)-sin(phi)*cos(psi); ...
           -sin(theta)    ,                sin(phi)*cos(theta)            ,                 cos(phi)*cos(theta)           ];

E_ro = Leb * B_vo;

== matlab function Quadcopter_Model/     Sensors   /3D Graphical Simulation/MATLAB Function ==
function y = eigenaxis_ucart(u)


if abs(u(1))< 0.0001
    u(1) = 0.0001;
end

if abs(u(2))< 0.0001
    u(2) = 0.0001;
end

if abs(u(3))< 0.0001
    u(3) = 0.0001;
end

u = [ -u(1); -u(2); u(3) ];% [Pitch, Yaw, Roll] 

C11 = cos(u(2))*cos(u(3));
C12 = cos(u(2))*sin(u(3));
C13 = -sin(u(2));
C21 = sin(u(1))*sin(u(2))*cos(u(3))-cos(u(1))*sin(u(3));
C22 = sin(u(1))*sin(u(2))*sin(u(3))+cos(u(1))*cos(u(3));
C23 = sin(u(1))*cos(u(2));
C31 = cos(u(1))*sin(u(2))*cos(u(3))+sin(u(1))*sin(u(3));
C32 = cos(u(1))*sin(u(2))*sin(u(3))-sin(u(1))*cos(u(3));
C33 = cos(u(1))*cos(u(2));
    
theta = acos(0.5*(C11+C22+C33-1));

e = [C23-C32; C31-C13; C12-C21]/(2*sin(theta));
    
y = [e; theta];

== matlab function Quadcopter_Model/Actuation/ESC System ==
function Vb_eff   = ESC(P, Pmin, Pmax, Vb)

P1 = P(1);
P2 = P(2);
P3 = P(3);
P4 = P(4);

% Define u_Pi for each of the rotors, limiting it to be greater than 0
u_P0 = (P1 - Pmin) / (Pmax - Pmin);
u_P1 = (P2 - Pmin) / (Pmax - Pmin);
u_P2 = (P3 - Pmin) / (Pmax - Pmin);
u_P3 = (P4 - Pmin) / (Pmax - Pmin);


% Determine the effective battery voltage from each ESC
Vb_eff_0 = u_P0 * Vb;
Vb_eff_1 = u_P1 * Vb;
Vb_eff_2 = u_P2 * Vb;
Vb_eff_3 = u_P3 * Vb;
    
Vb_eff = [Vb_eff_0, Vb_eff_1, Vb_eff_2, Vb_eff_3];

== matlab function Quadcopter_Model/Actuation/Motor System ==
function w_dot = motor(Vb_eff, w, Rm, Kv, Kq, Kd, If, Jreq)

% Define each motors effective battery voltage
Vb_eff_0 = Vb_eff(1);
Vb_eff_1 = Vb_eff(2);
Vb_eff_2 = Vb_eff(3);
Vb_eff_3 = Vb_eff(4);

% Determine the angular velocity of each rotor from feedback
w_0 = w(1);
w_1 = w(2);
w_2 = w(3);
w_3 = w(4);

% Determine angular acceleration of each rotor
w_0_dot = 1/(Jreq*Rm*Kq) * Vb_eff_0 - 1/(Jreq*Rm*Kq*Kv) * w_0 - 1/(Jreq*Kq)*If - (Kd/Jreq) * w_0^2;
w_1_dot = 1/(Jreq*Rm*Kq) * Vb_eff_1 - 1/(Jreq*Rm*Kq*Kv) * w_1 - 1/(Jreq*Kq)*If - (Kd/Jreq) * w_1^2;
w_2_dot = 1/(Jreq*Rm*Kq) * Vb_eff_2 - 1/(Jreq*Rm*Kq*Kv) * w_2 - 1/(Jreq*Kq)*If - (Kd/Jreq) * w_2^2;
w_3_dot = 1/(Jreq*Rm*Kq) * Vb_eff_3 - 1/(Jreq*Rm*Kq*Kv) * w_3 - 1/(Jreq*Kq)*If - (Kd/Jreq) * w_3^2;

w_dot = [w_0_dot, w_1_dot, w_2_dot, w_3_dot];

== matlab function Quadcopter_Model/Actuation/Rotor System







 ==
function [B_omega_dot, B_vo_dot]= rotor(w_dot, w, B_Fg, B_omega, B_vo, m, Kt, Kd, rhx, rhy, rhz, Jreq, Jxx, Jyy, Jzz, r_oc, Kh, delta_T)

% Create J vector
J = [Jxx,  0 ,  0 ; ...
      0 , Jyy,  0 ; ...
      0 ,  0 , Jzz;];
  
r_oc_X = [0, -r_oc(3), r_oc(2); r_oc(3), 0, -r_oc(1); -r_oc(2), r_oc(1), 0];

% Create r_hi vector
rh_0 = [-rhx; rhy; -rhz];
rh_1 = [rhx; rhy; -rhz];
rh_2 = [-rhx; -rhy; -rhz];
rh_3 = [rhx; -rhy; -rhz];

% Calculate rotor hub velocity
vh_0 = B_vo + cross(B_omega,rh_0);
vh_1 = B_vo + cross(B_omega,rh_1); 
vh_2 = B_vo + cross(B_omega,rh_2); 
vh_3 = B_vo + cross(B_omega,rh_3); 

% Define 3x3 Identity Matrix
I = eye(3);

% Create gamma vectors
gamma_Ti = [0; 0; -1];
gamma_omega_03 = [0; 0; 1];  %Rotors 0 and 3 use this gamma_omega vector
gamma_omega_12 = [0; 0; -1]; %Rotors 1 and 2 use this gamma_omega vector
gamma_Hi = [ 1 0 0 ; 0 1 0 ; 0 0 0 ];

% Define angular velocities for each rotor
w_0 = w(1);
w_1 = w(2);
w_2 = w(3);
w_3 = w(4);

% Define angular acceleration for each rotor
w_0_dot = w_dot(1);
w_1_dot = w_dot(2);
w_2_dot = w_dot(3);
w_3_dot = w_dot(4);

% Define the thrust force
T_0 = (Kt * w_0 * w_0 + delta_T * vh_0 * w_0) * gamma_Ti; 
T_1 = (Kt * w_1 * w_1 + delta_T * vh_1 * w_1) * gamma_Ti;
T_2 = (Kt * w_2 * w_2 + delta_T * vh_2 * w_2) * gamma_Ti;
T_3 = (Kt * w_3 * w_3 + delta_T * vh_3 * w_3) * gamma_Ti;

% Define the in plane drag force
H_0 = -Kh * w_0 * gamma_Hi * vh_0;
H_1 = -Kh * w_1 * gamma_Hi * vh_1;
H_2 = -Kh * w_2 * gamma_Hi * vh_2;
H_3 = -Kh * w_3 * gamma_Hi * vh_3;

% Define the rotor force in the z-direction from each rotor
B_Fr_0 = T_0 + H_0;
B_Fr_1 = T_1 + H_1;
B_Fr_2 = T_2 + H_2;
B_Fr_3 = T_3 + H_3;

% Sum up the rotor forces in the z-direction from each vector to get the
% total body force in the z-direction
B_Fr = B_Fr_0 + B_Fr_1 + B_Fr_2 + B_Fr_3;

% Define the in-plane drag and induced torque produced by each rotor
 B_Q_d0 = -1 * Kd * w_0 * w_0 * gamma_omega_03;
 B_Q_d1 = -1 * Kd * w_1 * w_1 * gamma_omega_12;
 B_Q_d2 = -1 * Kd * w_2 * w_2 * gamma_omega_12;
 B_Q_d3 = -1 * Kd * w_3 * w_3 * gamma_omega_03;

% Sum up the total in-plane drag and induced torque to get the total
% in-plane drag and induced torque on the body
B_Q_d = B_Q_d0 + B_Q_d1 + B_Q_d2 + B_Q_d3;

% Define the force lever arm torque created from the force produced by each
% rotor in the z-direction
B_Q_F0 = cross( rh_0, B_Fr_0 );
B_Q_F1 = cross( rh_1, B_Fr_1 );
B_Q_F2 = cross( rh_2, B_Fr_2 );
B_Q_F3 = cross( rh_3, B_Fr_3 );

B_Q_F = B_Q_F0 + B_Q_F1 + B_Q_F2 + B_Q_F3;

% Define the change in angular momentum torque produced by each rotor 
B_Q_L0 = -1 * Jreq * ( cross(B_omega, w_0 * gamma_omega_03) + w_0_dot * gamma_omega_03 );
B_Q_L1 = -1 * Jreq * ( cross(B_omega, w_1 * gamma_omega_12) + w_1_dot * gamma_omega_12 ); 
B_Q_L2 = -1 * Jreq * ( cross(B_omega, w_2 * gamma_omega_12) + w_2_dot * gamma_omega_12 ); 
B_Q_L3 = -1 * Jreq * ( cross(B_omega, w_3 * gamma_omega_03) + w_3_dot * gamma_omega_03 );

% Sum up the total change in angular momentum torque produced by each rotor
B_Q_L = B_Q_L0 + B_Q_L1 + B_Q_L2 + B_Q_L3;
    
% Define the total rotor system torque as the sum of the in-plane drag and
% induced torque, force lever arm torque, and change in angular momentum
% torques
B_Q = B_Q_d + B_Q_F + B_Q_L;

% Define the body forces in the z-direction from each vector to get the
% total body force in the z-direction
B_F = B_Fr + B_Fg; 

% Determine the dynamics of the system
M = [m * I , -m * r_oc_X; 
    zeros(3,3), J];

dynamics = M^-1*[B_F - m*cross(B_omega,B_vo) - m*cross(B_omega,cross(B_omega,r_oc)) ; ... 
          B_Q - cross(B_omega,J*B_omega) - cross(r_oc,B_F) ];

% Define the body frame angular velocities
B_vo_dot = dynamics(1:3);

% Define the body frame linear velocities
B_omega_dot = dynamics(4:6);

== matlab function Quadcopter_Model/Actuation/Aeb














 ==
function euler_rates = angular_body_earth_conversion(B_omega, euler_angles)

phi = euler_angles(1);
theta = euler_angles(2);

Aeb = [1,  sin(phi)*tan(theta), cos(phi)*tan(theta); ...
       0,      cos(phi)       ,        -sin(phi)   ; ...
       0,  sin(phi)/cos(theta), cos(phi)/cos(theta)];

   
euler_rates = Aeb * B_omega;

== matlab function Quadcopter_Model/Actuation/Lbe

















 ==
function [B_Fg, B_g]  = linear_earth_body_conversion(E_Fg, euler_angles, m)

phi = euler_angles(1);
theta = euler_angles(2);
psi = euler_angles(3);

Lbe = [             cos(theta)*cos(psi)              ,          cos(theta)*sin(psi)                  ,     -sin(theta)    ; ...
       sin(phi)*sin(theta)*cos(psi)-cos(phi)*sin(psi), sin(phi)*sin(theta)*sin(psi)+cos(phi)*cos(psi), sin(phi)*cos(theta); ...
       cos(phi)*sin(theta)*cos(psi)+sin(phi)*sin(psi), cos(phi)*sin(theta)*sin(psi)-sin(phi)*cos(psi), cos(phi)*cos(theta)];

B_Fg = Lbe * E_Fg;

B_g = B_Fg/m;

== matlab function Quadcopter_Model/     Sensors   /IMU





/






 ==
function [accelReading,gyroReading] = idealIMU(B_vo_dot, B_vo, B_Omega, B_g, g, r_oc)
%#codegen

a = B_vo_dot + cross(B_Omega,B_vo); % body frame acceleration 

accelReading = (a - B_g)/g ; % accelerometer reading (ideal)

gyroReading = B_Omega ; % gyroscope reading (ideal) 

end

== matlab function Quadcopter_Model/     Sensors   /Lbe





 ==
function B_vo  = linear_earth_body_conversion(E_vo, euler_angles)

phi = euler_angles(1);
theta = euler_angles(2);
psi = euler_angles(3);

Leb = [cos(theta)*cos(psi), sin(phi)*sin(theta)*cos(psi)-cos(phi)*sin(psi), cos(phi)*sin(theta)*cos(psi)+sin(phi)*sin(psi); ...
       cos(theta)*sin(psi), sin(phi)*sin(theta)*sin(psi)+cos(phi)*cos(psi), cos(phi)*sin(theta)*sin(psi)-sin(phi)*cos(psi); ...
           -sin(theta)    ,                sin(phi)*cos(theta)            ,                 cos(phi)*cos(theta)           ];

B_vo = Leb^-1 * E_vo;

== matlab function Quadcopter_Model/     Sensors   /Aeb









 ==
function euler_rates_IMU = angular_body_earth_conversion(gyro_reading, euler_angles_filtered)

phi = euler_angles_filtered(1);
theta = euler_angles_filtered(2);

Aeb = [1, sin(phi)*tan(theta), cos(phi)*tan(theta); ...
       0,     cos(phi)       ,        -sin(phi)   ; ...
       0,  sin(phi)/cos(theta), cos(phi)/cos(theta)];

   
euler_rates_IMU = Aeb * gyro_reading;

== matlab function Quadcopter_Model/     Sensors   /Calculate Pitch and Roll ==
function [accel_pitch, accel_roll] = getPitchAndRoll(accel_reading)

x_accel = accel_reading(1);
y_accel = accel_reading(2);
z_accel = accel_reading(3);

accel_pitch = atan(x_accel/sqrt(y_accel^2 + z_accel^2));
accel_roll = atan( -y_accel/( sqrt(z_accel^2 + x_accel^2))  );

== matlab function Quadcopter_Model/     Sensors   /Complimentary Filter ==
function euler_angles_IMU   = complimentaryFilter(accel_pitch, accel_roll, euler_rates_gyro, prev_euler_angles)

k_gyro = 0.99; 
k_accel = 1-k_gyro; 

Ts = 0.005; % 5 milliseconds

prev_phi = prev_euler_angles(1);
prev_theta = prev_euler_angles(2);

prev_phi_dot = euler_rates_gyro(1);
prev_theta_dot = euler_rates_gyro(2);

integrated_phi_gyro = Ts * prev_phi_dot + prev_phi;
integrated_theta_gyro = Ts * prev_theta_dot + prev_theta;

phi = k_gyro * integrated_phi_gyro + k_accel * accel_roll;
theta = k_gyro * integrated_theta_gyro + k_accel * accel_pitch;

euler_angles_IMU = [phi; theta];
